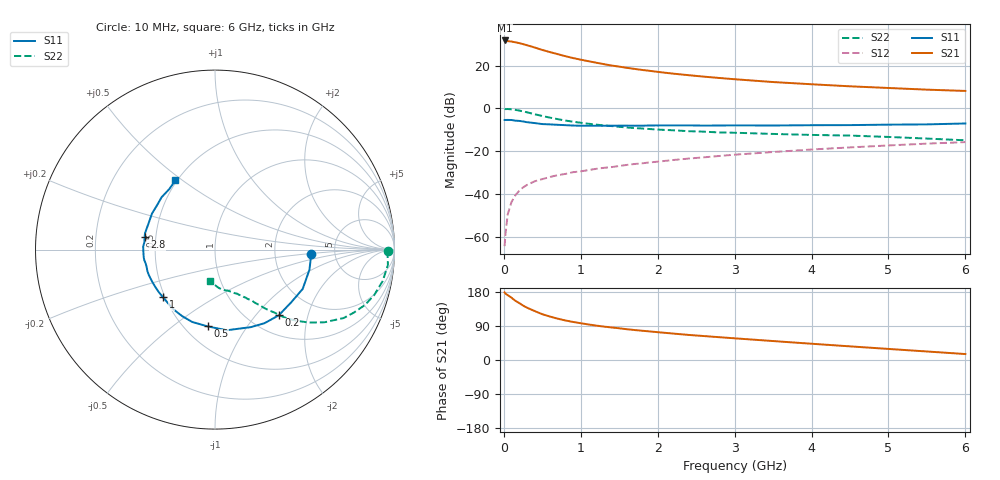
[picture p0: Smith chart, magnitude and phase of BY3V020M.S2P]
! SIEMENS Small Signal Semiconductors
! BFY420
! Si NPN RF SIEGET Grounded Emitter Transistor in MICRO-X
! VCE = 3 V  IC = 20 mA
! Common Emitter S-Parameters:  October  1996
# GHz  S  MA  R  50
!  f  S11  S21  S12  S22
! GHz  MAG  ANG  MAG  ANG  MAG  ANG  MAG  ANG
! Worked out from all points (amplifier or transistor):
!   36 points, 10 MHz to 6 GHz, reference 50 ohm
!   highest |S21| = 31.8 dB at 10 MHz (marker M1)
!   |S21| within 3 dB of that: start of sweep to 373.2 MHz
!   unconditionally stable (mu >= 1): 1.973 GHz to end of sweep
!   at 250 MHz: K = 0.30, MSG = 33.5 dB, |S12| = -37.0 dB
!   at 1.4 GHz: K = 0.91, MSG = 23.8 dB, |S12| = -27.5 dB
!   at 6 GHz: K = 1.07, MAG = 10.4 dB, |S12| = -15.8 dB
!   S11 on the Smith chart (normalised r, x): 10 MHz: 3.29, -0.22; 200 MHz: 1.34, -1.33; 500 MHz: 0.64, -0.68; 1 GHz: 0.49, -0.31; 2.8 GHz: 0.43, +0.07; 6 GHz: 0.49, +0.47
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0.01  0.5357 -2.5  38.79 178.4  0.0006 108.7  0.9632 -0.4
0.02  0.5362 -5.1  38.62 175.5  0.0011 84.5  0.962 -1.5
0.05  0.5379 -12.1  37.38 171.2  0.0033 81.6  0.9672 -5.1
0.1  0.5355 -24.1  36.6 164.3  0.0065 80.3  0.9502 -10.7
0.15  0.5161 -34.8  35.11 156.2  0.0093 73.7  0.923 -15.8
0.2  0.5102 -45.9  33.68 150.3  0.0118 73.2  0.8907 -20.3
0.25  0.4941 -56.1  31.86 143.6  0.0142 68.2  0.8484 -24.5
0.3  0.4759 -65.2  30.07 138.1  0.0162 67.3  0.8119 -28.0
0.4  0.4541 -81.7  26.56 129.2  0.0197 62.8  0.7318 -33.6
0.5  0.4298 -95.5  23.26 120.8  0.0222 59.9  0.6637 -37.8
0.6  0.4227 -107.5  20.71 114.6  0.0249 59.0  0.6079 -40.8
0.7  0.4132 -116.4  18.57 109.1  0.0274 58.3  0.5607 -43.4
0.8  0.4054 -124.6  16.63 104.4  0.0294 57.8  0.5202 -45.2
1  0.3931 -137.4  13.77 97.0  0.0337 58.0  0.4617 -47.8
1.1  0.3927 -143.4  12.69 93.8  0.0361 58.2  0.4383 -49.2
1.6  0.3953 -162.5  8.872 81.2  0.0477 58.4  0.3571 -53.8
2.2  0.3993 -178.1  6.497 69.8  0.062 57.3  0.3077 -58.8
2.8  0.3981 170.1  5.143 60.2  0.0771 54.4  0.2741 -63.5
3.5  0.3981 158.0  4.135 50.0  0.0955 50.1  0.2528 -68.8
4.5  0.4065 142.6  3.284 36.0  0.1224 42.5  0.2313 -77.4
5.5  0.4227 127.0  2.743 22.5  0.15 33.6  0.1969 -90.4
6  0.4442 119.9  2.56 15.7  0.1627 28.7  0.1794 -99.1
